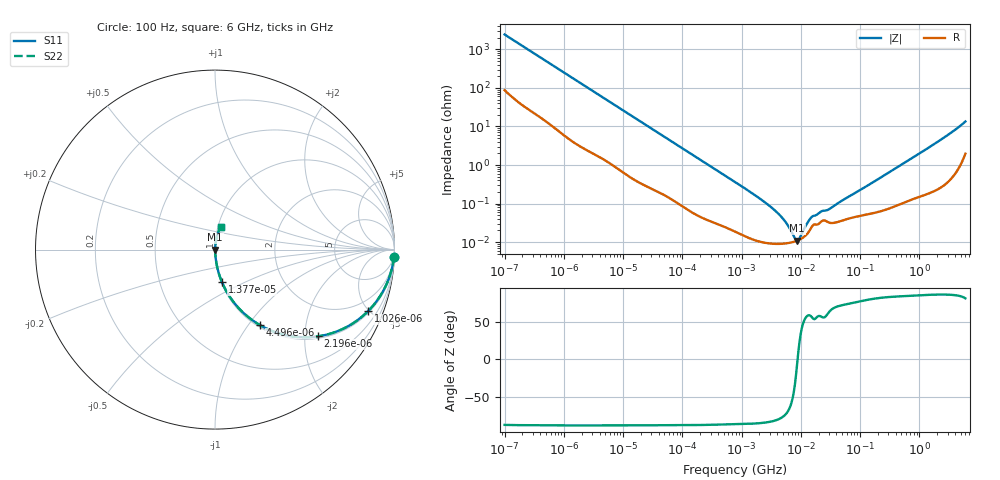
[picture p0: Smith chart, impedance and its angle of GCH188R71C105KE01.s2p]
!Murata Part Number: GCH188R71C105KE01
!These Parameters are Measured in Series Mode Connection
!Data Generated on Mar 13, 2026
!  o--ll--o
!Port1  Port2
!  o------o
!Operation Temp=25[degC], DC Bias Voltage=0[V]
!Freq. Start=100[Hz] Stop=6[GHz] 401[Steps]
# Hz S RI R 50
!Freq.(Hz) S11(Real) S11(Imag) S21(Real) S21(Imag) S12(Real) S12(Imag) S22(Real) S22(Imag)
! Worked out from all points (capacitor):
!   401 points, 100 Hz to 6 GHz, reference 50 ohm
!   read as one part in series: C = 650 nF near 109 Hz
!   lowest |Z| = 10.9 mohm at 8.692 MHz (marker M1)
!   series resonance near 8.827 MHz, so ESL is about 500 pH
!   S11 on the Smith chart (normalised r, x): 100 Hz: 3, -49; 1.026 kHz: 1.11, -4.92; 2.196 kHz: 1.05, -2.32; 4.496 kHz: 1.03, -1.15; 13.77 kHz: 1.01, -0.38; 6 GHz: 1.04, +0.27
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100  0.9969 -0.0408  0.00314 0.0408  0.00314 0.0408  0.9969 -0.0408
350  0.9768 -0.1373  0.0232 0.1373  0.0232 0.1373  0.9768 -0.1373
1026  0.8526 -0.3431  0.1474 0.3431  0.1474 0.3431  0.8526 -0.3431
2008  0.6136 -0.4758  0.3864 0.4758  0.3864 0.4758  0.6136 -0.4758
2196  0.5718 -0.4835  0.4282 0.4835  0.4282 0.4835  0.5718 -0.4835
4496  0.2524 -0.4219  0.7476 0.4219  0.7476 0.4219  0.2524 -0.4219
7358  0.1169 -0.309  0.8831 0.309  0.8831 0.309  0.1169 -0.309
13772  0.0391 -0.182  0.9609 0.182  0.9609 0.182  0.0391 -0.182
40335  0.00627 -0.0655  0.9937 0.0655  0.9937 0.0655  0.00627 -0.0655
774597  0.0002 -0.00362  0.9998 0.00362  0.9998 0.00362  0.0002 -0.00362
2074311  0.000103 -0.00131  0.9999 0.00131  0.9999 0.00131  0.000103 -0.00131
3712478  9.02e-05 -0.000642  0.9999 0.000642  0.9999 0.000642  9.02e-05 -0.000642
5311619  9.16e-05 -0.000349  0.9999 0.000349  0.9999 0.000349  9.16e-05 -0.000349
7947587  0.000104 -6.97e-05  0.9999 6.97e-05  0.9999 6.97e-05  0.000104 -6.97e-05
8692127  0.000109 -1.01e-05  0.9999 1.01e-05  0.9999 1.01e-05  0.000109 -1.01e-05
9506416  0.000116 4.98e-05  0.9999 -4.98e-05  0.9999 -4.98e-05  0.000116 4.98e-05
1.300572e7  0.000168 0.000272  0.9998 -0.000272  0.9998 -0.000272  0.000168 0.000272
1.555665e7  0.000258 0.00038  0.9997 -0.00038  0.9997 -0.00038  0.000258 0.00038
3.045065e7  0.000319 0.00065  0.9997 -0.00065  0.9997 -0.00065  0.000319 0.00065
3.124326e8  0.000788 0.00647  0.9992 -0.00647  0.9992 -0.00647  0.000788 0.00647
1.95892e9  0.0037 0.0381  0.9963 -0.0381  0.9963 -0.0381  0.0037 0.0381
6e9  0.0357 0.1261  0.9643 -0.1261  0.9643 -0.1261  0.0357 0.1261
